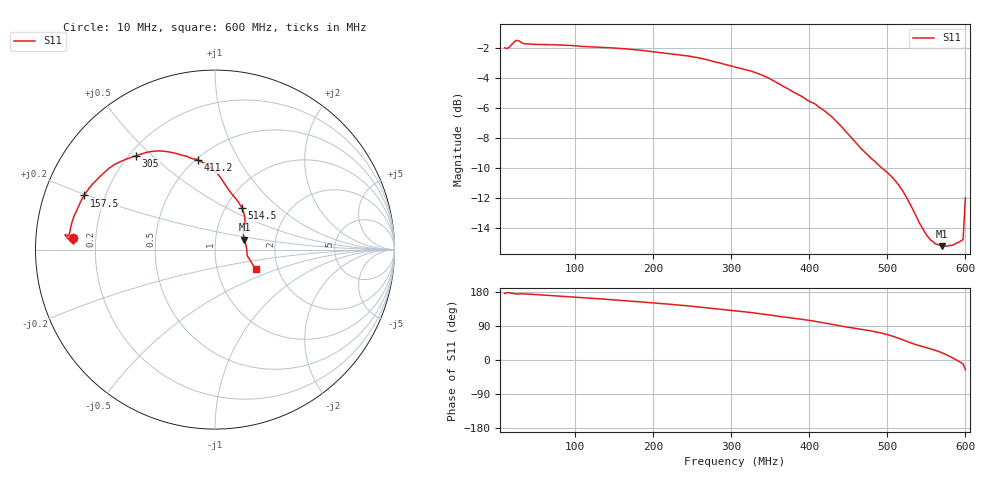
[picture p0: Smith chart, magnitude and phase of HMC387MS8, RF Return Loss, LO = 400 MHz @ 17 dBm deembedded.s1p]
!Hittite Microwave Corporation
!12 Elizabeth Drive
!Chelmsford, MA 01824
!Tel: 978-250-3343
!Fax: 978-250-3373
!Device: HMC387MS8, 450-500 MHz, GaAs MMIC High IP3 Mixer in 8-lead plastic SMT package
!Misc: RF Return Loss, LO = 400 MHz @ 17 dBm, Room
# MHZ S MA R 50
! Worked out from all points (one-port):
!   201 points, 10 MHz to 600 MHz, reference 50 ohm
!   lowest |S11| = -15.2 dB at 570.5 MHz (marker M1), VSWR 1.42, Z = 69.1 + j7.85 ohm
!   |S11| at or under -10 dB: 492.5 MHz to end of sweep
!   S11 on the Smith chart (normalised r, x): 10 MHz: 0.12, +0.04; 157.5 MHz: 0.12, +0.20; 305 MHz: 0.23, +0.44; 411.2 MHz: 0.52, +0.69; 514.5 MHz: 1.19, +0.60; 600 MHz: 1.53, -0.36
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10  0.793 175.4
12.95  0.788 177.8
15.9  0.797 177.3
24.75  0.839 174.4
33.6  0.82 174.5
83.75  0.81 168.2
157.5  0.789 157.5
192.9  0.774 151.9
231.25  0.752 145.4
263.7  0.729 138.8
305  0.684 130.2
325.65  0.663 125.3
346.3  0.632 119.5
378.75  0.567 110.6
411.2  0.506 100.7
428.9  0.467 94.2
452.5  0.402 85.6
467.25  0.364 80.9
499.7  0.305 67.3
514.45  0.277 57.4
526.25  0.247 48.1
541  0.207 37.8
549.85  0.189 32.7
561.65  0.176 25.5
570.5  0.173 18.6
582.3  0.174 7.0
597.05  0.182 -10.4
600  0.251 -25.8
